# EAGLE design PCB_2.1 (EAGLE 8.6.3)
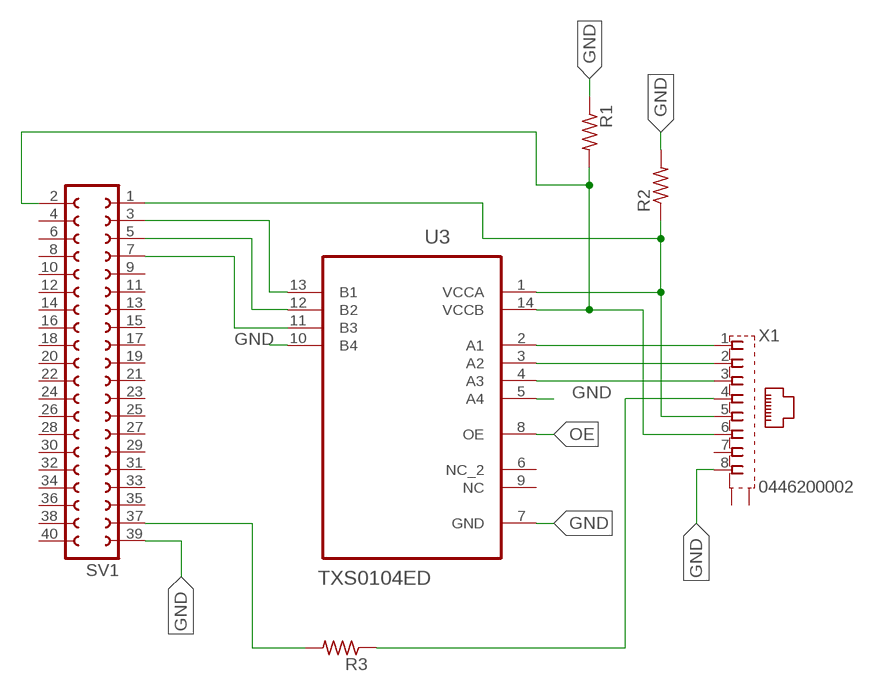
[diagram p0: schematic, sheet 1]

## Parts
R1  R-US_R0805  [R0805]
R2  R-US_R0805  [R0805]
R3  R-US_R0805  [R0805]
SV1  FE20-2  [FE20-2]
U3  TXS0104ED  [SOIC127P600X175-14N]
X1  0446200002  [0446200002]

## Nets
A1: U3.2(A1) X1.1
A2: U3.3(A2) X1.2
A3: U3.4(A3) X1.3
GND: R1.1 R2.2 SV1.39 U3.5(A4) U3.7(GND) U3.10(B4) X1.8
INT: SV1.7 U3.11(B3)
LED: R3.1 X1.4
N$1: R3.2 SV1.37
OE: U3.8(OE)
SCL: SV1.5 U3.12(B2)
SDA: SV1.3 U3.13(B1)
VCCA: R2.1 SV1.1 U3.1(VCCA) X1.5
VCCB: R1.2 SV1.2 U3.14(VCCB) X1.6
Unconnected: SV1.4 SV1.6 SV1.8 SV1.9 SV1.10 SV1.11 SV1.12 SV1.13 SV1.14 SV1.15 SV1.16 SV1.17 SV1.18 SV1.19 SV1.20 SV1.21 SV1.22 SV1.23 SV1.24 SV1.25 SV1.26 SV1.27 SV1.28 SV1.29 SV1.30 SV1.31 SV1.32 SV1.33 SV1.34 SV1.35 SV1.36 SV1.38 SV1.40 U3.6(NC_2) U3.9(NC) X1.7 X1.S@1(S1) X1.S@2(S2)

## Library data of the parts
R1-R3 = resistor:R-US_: RESISTOR, American symbol
SV1 = con-lsta:FE20-2: FEMALE HEADER; OC_FARNELL: unknown; OC_NEWARK: unknown
U3 = TXS0104ED:TXS0104ED: 4-BIT BIDIRECTIONAL VOLTAGE-LEVEL TRANSLATOR FOR OPEN-DRAIN AND PUSH-PULL APPLICATIONS; AVAILABILITY: Unavailable; DESCRIPTION: 4-Bit Bidirectional Voltage-Level Shifter for Open-Drain and Push-Pull Applications 14-SOIC -40 to 85; MF: Texas Instruments; MP: TXS0104ED; PACKAGE: SOIC-14 Texas Instruments; PRICE: None
X1 = 0446200002:0446200002: RJ-45 INVERTED MODULAR JACK ASSEMBLY WITH RJ-11 KEEPOUT FEATURE Source: Data sheet MOLEX 0446200002 BUCHSE, RJ45, GESCHIRMT Source: Farnell; AVAILABILITY: Unavailable; DESCRIPTION: Conn RJ-45 RCP 8 POS 2.04mm Solder RA Thru-Hole 8 Terminal 1 Port Tray Cat 3; MF: Molex, LLC; MP: 0446200002; PACKAGE: None; PRICE: None

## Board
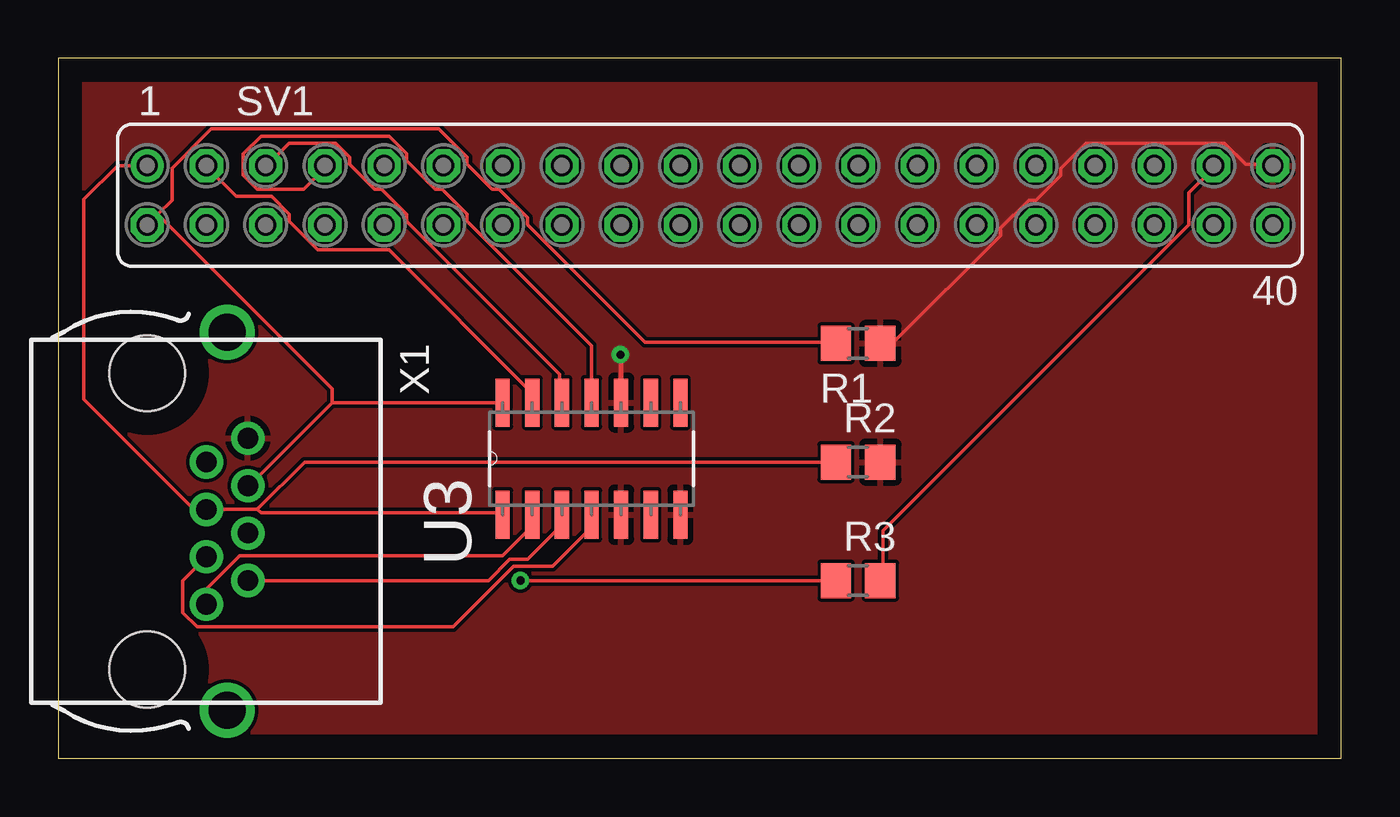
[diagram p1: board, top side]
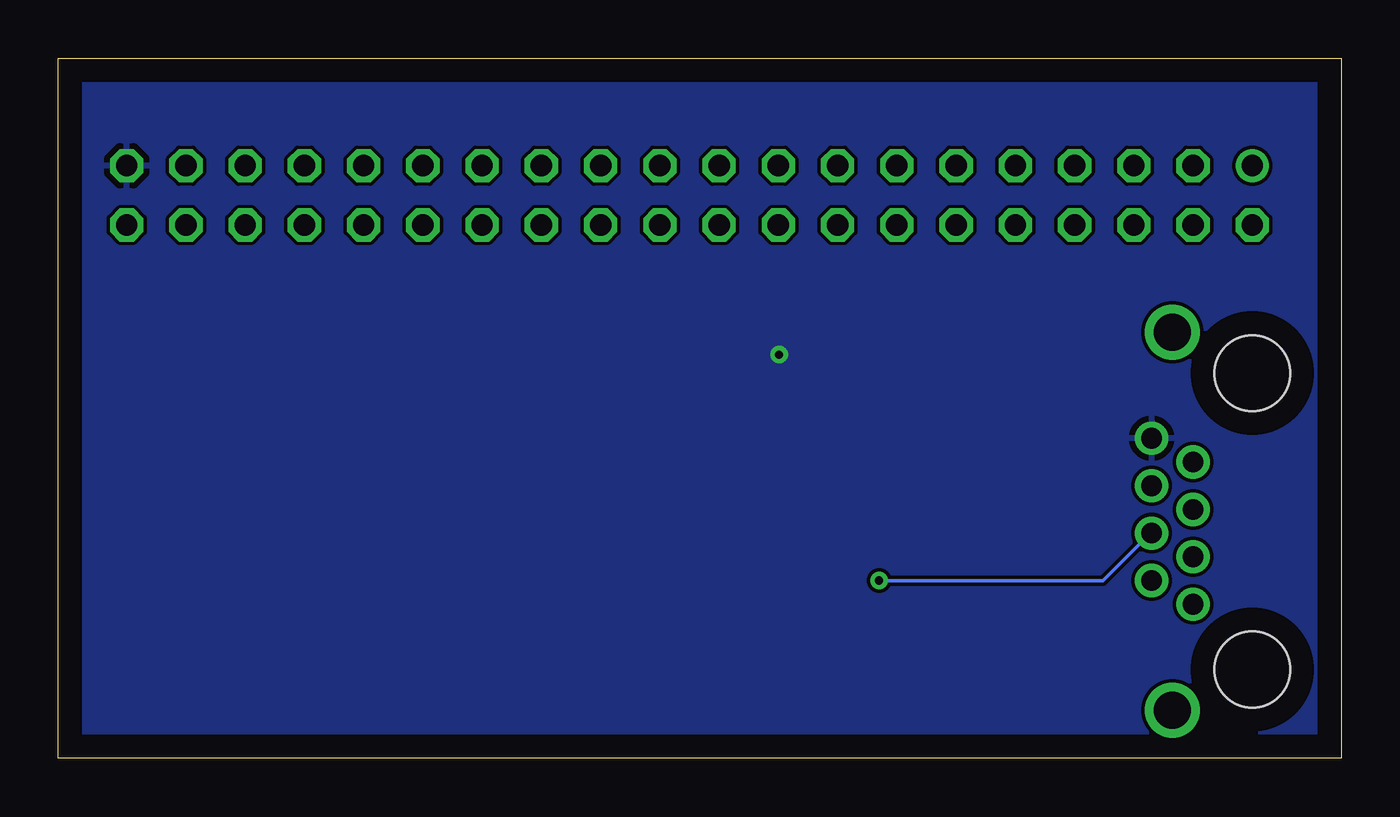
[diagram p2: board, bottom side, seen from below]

Size 55 x 30 mm. Coordinates in mm from the lower left corner, seen from the top.
Outline: 0,0 55,0 55,30 0,30 0,0
Copper layers (1*16): Top 0.035mm / dielectric 1.5mm / Bottom 0.035mm
Design rules "default *": minimum track width 6mil, minimum drill 0.35mm, track to track 6mil, track to pad 6mil, pad to pad 6mil, via to via 6mil, smd to smd 6mil, copper to edge 40mil, drill to drill 6mil, minimum pad ring 10mil, minimum via ring 8mil, stop-mask expansion 4mil, vias tented up to drill 0mil, thermal gap 10mil

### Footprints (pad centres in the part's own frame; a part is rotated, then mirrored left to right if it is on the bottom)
R0805 = smd 1.3 x 1.5: 1 -0.95,0; 2 0.95,0
FE20-2 = drill 0.914: 1 -24.13,1.27 | drill 0.914 octagon: 2 -24.13,-1.27; 3 -21.59,1.27; 4 -21.59,-1.27; 5 -19.05,1.27; 6 -19.05,-1.27; 7 -16.51,1.27; 8 -16.51,-1.27; 9 -13.97,1.27; 10 -13.97,-1.27; 11 -11.43,1.27; 12 -11.43,-1.27; 13 -8.89,1.27; 14 -8.89,-1.27; 15 -6.35,1.27; 16 -6.35,-1.27; 17 -3.81,1.27; 18 -3.81,-1.27; 19 -1.27,1.27; 20 -1.27,-1.27; 21 1.27,1.27; 22 1.27,-1.27; 23 3.81,1.27; 24 3.81,-1.27; 25 6.35,1.27; 26 6.35,-1.27; 27 8.89,1.27; 28 8.89,-1.27; 29 11.43,1.27; 30 11.43,-1.27; 31 13.97,1.27; 32 13.97,-1.27; 33 16.51,1.27; 34 16.51,-1.27; 35 19.05,1.27; 36 19.05,-1.27; 37 21.59,1.27; 38 21.59,-1.27; 39 24.13,1.27; 40 24.13,-1.27
SOIC127P600X175-14N = smd 2.057 x 0.61: 1 -4.801,7.62; 2 -4.801,6.35; 3 -4.801,5.08; 4 -4.801,3.81; 5 -4.801,2.54; 6 -4.801,1.27; 7 -4.801,0; 8 0,0; 9 0,1.27; 10 0,2.54; 11 0,3.81; 12 0,5.08; 13 0,6.35; 14 0,7.62
0446200002 = drill 0.889 pad 1.422: 1 3.556,2.54; 2 2.54,4.318; 3 1.524,2.54; 4 0.508,4.318; 5 -0.508,2.54; 6 -1.524,4.318; 7 -2.54,2.54; 8 -3.556,4.318 | drill 1.575 pad 2.286: S@1 -8.103,3.429; S@2 8.103,3.429 | hole 3.251: 6.35,0; -6.35,0

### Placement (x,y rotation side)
R1  34.29,17.78 180 top
R2  34.29,12.7 0 top
R3  34.29,7.62 0 top
SV1  27.94,24.13 0 top
U3  26.67,15.24 90 top
X1  3.81,10.16 270 top

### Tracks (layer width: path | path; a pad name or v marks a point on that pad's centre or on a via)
A1
  Top 0.152: U3.2 20.27,10.36 20.27,9.91 19.05,8.69 7.77,8.69 6.4,7.32 6.4,6.71 X1.1
A2
  Top 0.152: X1.2 18.44,7.62 19.36,8.53 20.12,8.53 21.49,9.91 21.49,10.36 U3.3
A3
  Top 0.152: U3.4 22.86,9.91 21.18,8.23 19.51,8.23 16.92,5.64 5.94,5.64 5.33,6.25 5.33,7.62 X1.3
GND  (via drill 0.35)
  Top 0.152: SV1.39 51.97,25.45 50.9,25.45 49.99,26.36 44.04,26.36 42.98,25.3 42.98,24.99 41.91,23.93 41.6,23.93 40.39,22.71 40.39,22.4 35.81,17.83 35.36,17.83 R1.1
  Top 0.203: 24.1,17 24.13,17 U3.10
  other vias: 24.1,17.3
  pour Top: 0,30 55.4,30 55.4,0.1 0,0.1
  pour Bottom: 0,29.9 0,0 55.4,0 55.4,29.9
INT
  Top 0.152: U3.11 22.86,17.68 17.53,23.01 17.53,23.32 16.46,24.38 16.15,24.38 14.94,25.6 14.94,25.91 14.17,26.67 8.69,26.67 7.92,25.91 7.92,24.99 8.53,24.38 10.52,24.38 11.43,25.3 SV1.7
LED  (via drill 0.35)
  Top 0.152: v19.81,7.62 R3.1
  Bottom 0.152: v19.81,7.62 10.21,7.62 8.23,9.6 X1.4
N$1
  Top 0.152: R3.2 35.36,7.62 35.36,9.75 48.46,22.86 48.46,24.23 49.53,25.3 SV1.37
SCL
  Top 0.152: U3.12 21.49,15.24 21.49,16.46 14.94,23.01 14.94,23.32 13.87,24.38 13.56,24.38 12.5,25.45 12.5,25.76 11.89,26.36 9.91,26.36 8.99,25.45 SV1.5
SDA
  Top 0.152: U3.13 20.27,15.24 20.27,15.7 14.17,21.79 11.12,21.79 9.91,23.01 9.91,23.32 9.14,24.08 7.62,24.08 6.4,25.3 SV1.3
VCCA
  Top 0.152: 8.53,10.67 8.69,10.52 19.05,10.52 U3.1 | 8.53,10.67 X1.5 5.81,10.67 1.09,15.38 1.09,23.95 2.54,25.4 SV1.1 | R2.1 10.57,12.7 8.53,10.67
VCCB
  Top 0.152: 11.73,15.24 U3.14 | 11.73,15.24 8.23,11.73 X1.6 | 4.27,23.32 4.88,23.93 4.88,25.3 6.55,26.98 16.31,26.98 17.53,25.76 17.53,25.45 18.59,24.38 18.9,24.38 20.12,23.16 20.12,22.86 25.15,17.83 33.22,17.83 R1.2 | 11.73,15.24 11.73,15.85 4.27,23.32 | 4.27,23.32 SV1.2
